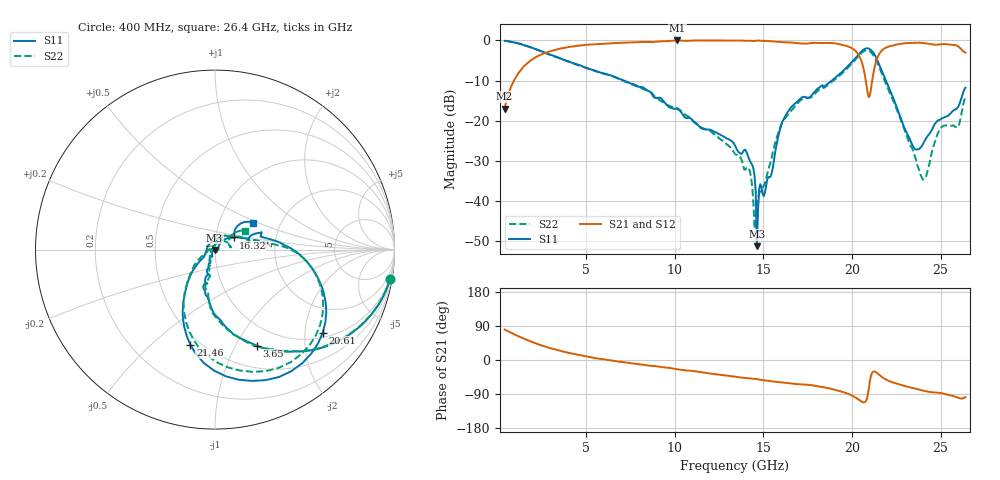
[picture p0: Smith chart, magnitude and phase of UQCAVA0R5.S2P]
!  Part Number  UQCAVA0R5  Mounting Orientation: Horizontal
!  Description: Ultra Low ESR Microwave capacitors
!  Application: Coupling, Bypass, Tuning, DC Block
!  Filters, Matching
# GHZ S DB R 50
! Freq  |S11|  S11 Ph  |S21|  S21 Ph  |S12|  S12 Ph  |S22|  S22 Ph
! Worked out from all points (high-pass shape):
!   401 points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, 400 MHz to 26.4 GHz, reference 50 ohm
!   highest |S21| = 0.00 dB at 10.15 GHz (marker M1); lowest = -16.9 dB at 400 MHz (marker M2)
!   |S21| within 3 dB of the highest: 2.747 GHz to 20.28 GHz (17.53 GHz wide, 152 % of centre); 21.59 GHz to 26.39 GHz (4.794 GHz wide, 20 % of centre)
!   lowest |S11| = -51.2 dB at 14.63 GHz (marker M3), VSWR 1.01, Z = 49.8 - j0.131 ohm
!   |S11| at or under -10 dB: 7.148 GHz to 18.86 GHz (11.71 GHz wide, 90.1 % of centre); 21.91 GHz to end of sweep
!   |S22| runs from -46.9 to -0.1 dB; largest |S21 - S12| = 0.0021
!   S11 on the Smith chart (normalised r, x): 400 MHz: 1, -12; 3.65 GHz: 0.75, -1.22; 16.32 GHz: 1.22, +0.17; 20.61 GHz: 1.13, -2.48; 21.46 GHz: 0.44, -0.68; 26.4 GHz: 1.45, +0.47
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0.4  -0.09 -9.5  -16.94 80.3  -16.93 80.3  -0.09 -9.6
1.505  -1.15 -33.8  -6.39 56.0  -6.38 55.9  -1.17 -33.8
3.65  -4.67 -66.6  -1.92 22.9  -1.92 22.8  -4.68 -66.7
4.755  -6.39 -78.2  -1.21 11.6  -1.21 11.6  -6.49 -78.5
9.11  -14.26 -103.1  -0.23 -17.4  -0.23 -17.4  -14.75 -104.4
10.15  -17.04 -106.0  0.00 -24.6  -0.01 -24.6  -16.85 -102.2
13.4  -26.13 -125.5  -0.01 -44.1  -0.01 -44.1  -28.22 -132.4
14.31  -30.52 -121.9  -0.10 -49.2  -0.10 -49.3  -34.18 173.5
14.635  -51.18 -151.6  -0.05 -50.4  -0.06 -50.4  -40.59 -148.2
15.415  -33.80 20.4  -0.18 -55.9  -0.19 -55.9  -30.15 89.2
16.325  -18.18 33.2  -0.48 -60.5  -0.49 -60.6  -18.79 40.0
17.755  -13.52 21.0  -0.62 -66.7  -0.62 -66.7  -13.96 12.9
19.77  -6.38 -4.0  -1.48 -89.0  -1.48 -88.9  -6.77 -2.6
20.615  -2.40 -37.7  -6.32 -111.4  -6.32 -111.3  -2.85 -35.5
21.005  -2.16 -68.9  -13.79 -57.3  -13.78 -57.4  -2.69 -67.4
21.46  -5.21 -104.4  -4.05 -36.1  -4.06 -36.2  -5.81 -103.9
22.11  -11.96 -128.4  -1.47 -55.9  -1.47 -55.9  -12.85 -131.5
23.475  -26.60 -178.0  -0.61 -74.5  -0.61 -74.5  -27.79 -169.8
24.06  -25.26 92.8  -0.65 -81.4  -0.65 -81.4  -34.57 115.6
24.905  -19.80 47.4  -1.02 -86.4  -1.02 -86.4  -22.55 37.0
25.945  -16.80 41.7  -1.36 -99.0  -1.36 -99.0  -21.64 19.6
26.4  -11.73 35.5  -3.03 -98.1  -3.03 -98.1  -14.02 32.0
